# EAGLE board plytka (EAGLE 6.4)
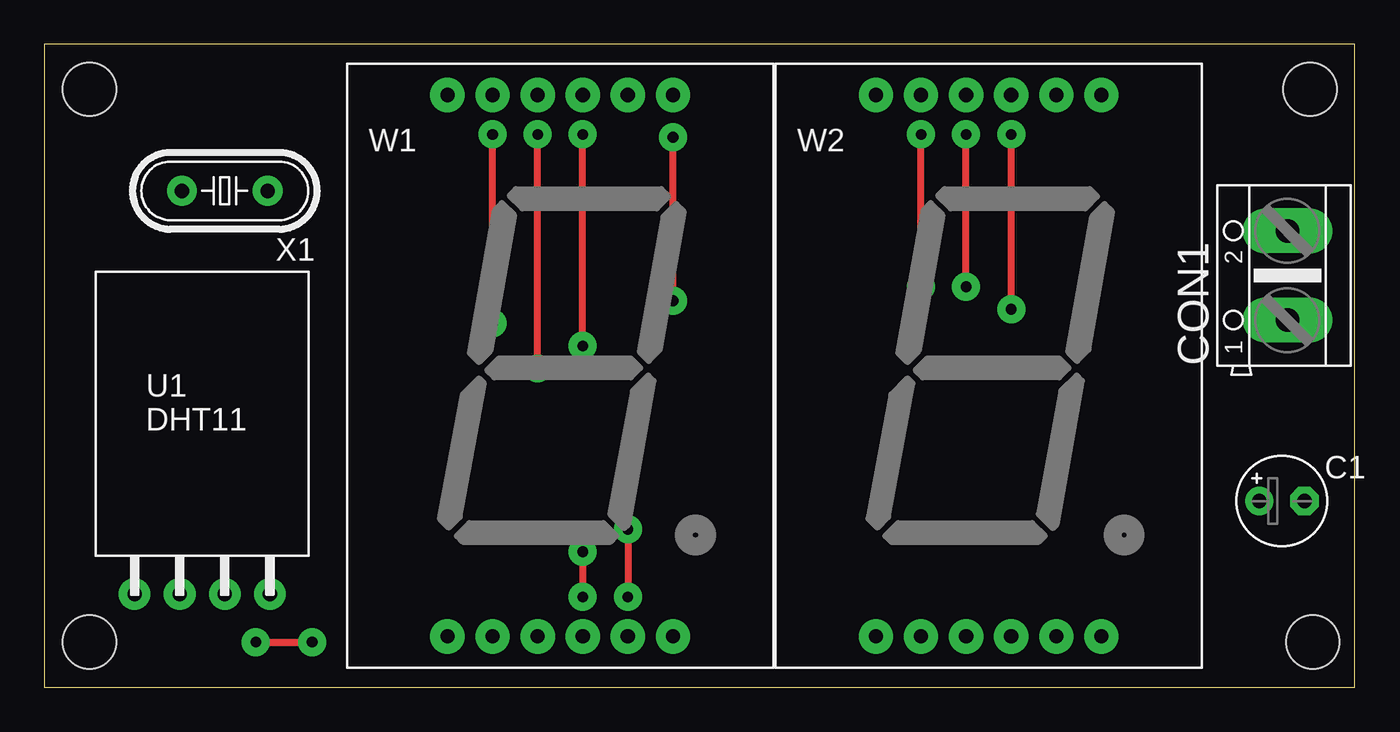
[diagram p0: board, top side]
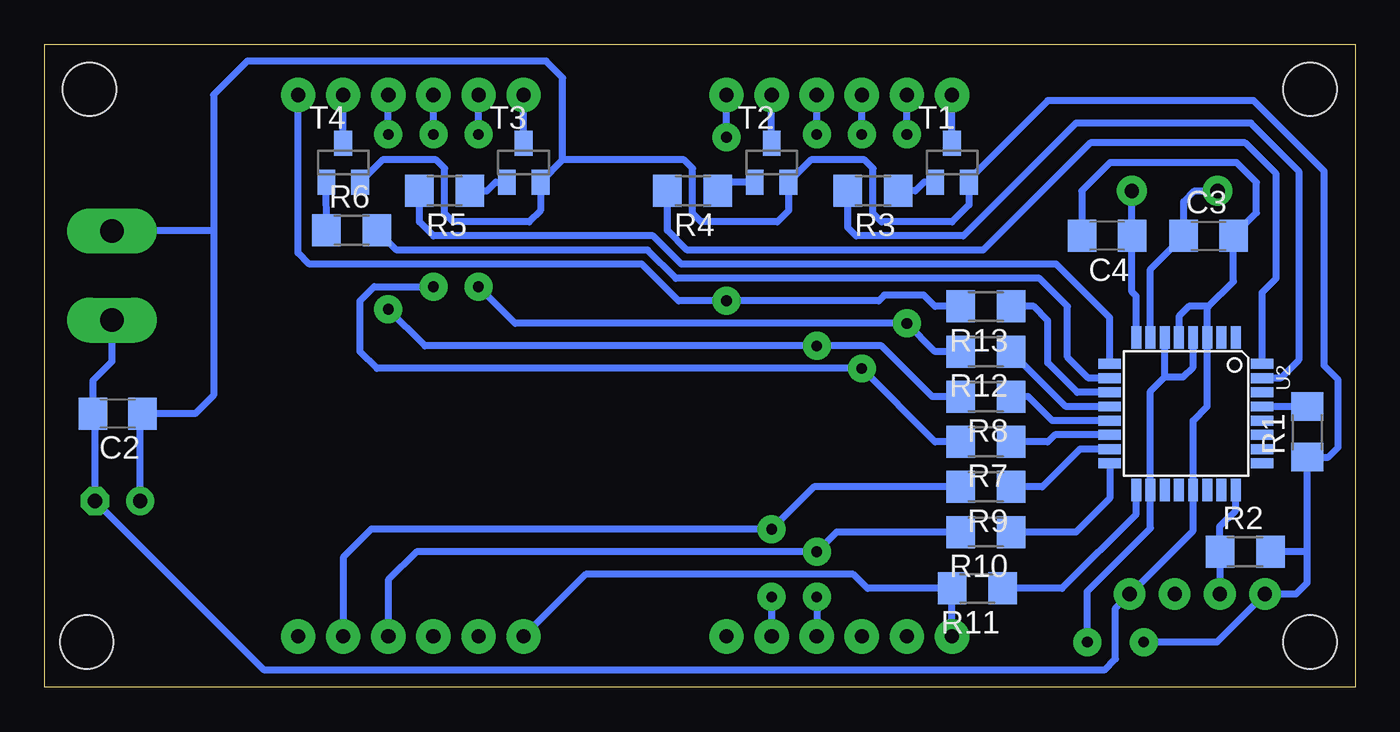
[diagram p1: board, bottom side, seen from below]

Size 73.81 x 36.19 mm. Coordinates in mm from the lower left corner, seen from the top.
Outline: 0,0 73.81,0 73.81,36.19 0,36.19 0,0
Copper layers (1*16): Top 0.035mm / dielectric 1.5mm / Bottom 0.035mm
Design rules "default": minimum track width 10mil, minimum drill 24mil, track to track 8mil, track to pad 8mil, pad to pad 8mil, via to via 8mil, smd to smd 8mil, copper to edge 40mil, drill to drill 8mil, minimum pad ring 10mil, minimum via ring 8mil, stop-mask expansion 4mil, vias tented up to drill 0mil, thermal gap 10mil
Holes 3 mm at 71.28,33.66 71.44,2.54 2.54,33.66 2.54,2.54

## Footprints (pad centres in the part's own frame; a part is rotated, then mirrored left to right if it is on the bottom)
E2,5-5 = drill 0.813 pad 1.6: + -1.27,0 | drill 0.813 pad 1.6 octagon: - 1.27,0
C1206 = smd 1.6 x 1.8: 1 -1.4,0; 2 1.4,0
AK500/2 = drill 1.321 pad 2.54 long: 1 -2.515,0; 2 2.515,0
R1206 = smd 1.6 x 1.803: 1 -1.422,0; 2 1.422,0
SOT23-BEC = smd 1 x 1.4: B -0.95,-1.1; C 0,1.1; E 0.95,-1.1
DHT11 = drill 0.8 pad 1.778: 1 -3.81,-10.16; 2 -1.27,-10.16; 3 1.27,-10.16; 4 3.81,-10.16
TQFP32-08 = smd 1.27 x 0.559: 1 -4.293,2.8; 2 -4.293,2; 3 -4.293,1.2; 4 -4.293,0.4; 5 -4.293,-0.4; 6 -4.293,-1.2; 7 -4.293,-2; 8 -4.293,-2.8; 17 4.293,-2.8; 18 4.293,-2; 19 4.293,-1.2; 20 4.293,-0.4; 21 4.293,0.4; 22 4.293,1.2; 23 4.293,2; 24 4.293,2.8 | smd 0.559 x 1.27: 9 -2.8,-4.293; 10 -2,-4.293; 11 -1.2,-4.293; 12 -0.4,-4.293; 13 0.4,-4.293; 14 1.2,-4.293; 15 2,-4.293; 16 2.8,-4.293; 25 2.8,4.293; 26 2,4.293; 27 1.2,4.293; 28 0.4,4.293; 29 -0.4,4.293; 30 -1.2,4.293; 31 -2,4.293; 32 -2.8,4.293
LED1-AS-10016 = drill 0.8 pad 1.93: 1 -6.35,-15.24; 2 -3.81,-15.24; 3 -1.27,-15.24; 4 1.27,-15.24; 5 3.81,-15.24; 6 6.35,-15.24; 7 6.35,15.24; 8 3.81,15.24; 9 1.27,15.24; 10 -1.27,15.24; 11 -3.81,15.24; 12 -6.35,15.24
HC49/S = drill 0.813 pad 1.676: 1 -2.413,0; 2 2.413,0

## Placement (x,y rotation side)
C1  10u  [E2,5-5]  69.69,10.48 0 top
C2  100n  [C1206]  69.69,15.4 180 bottom
C3  33p  [C1206]  8.26,25.4 0 bottom
C4  33p  [C1206]  13.97,25.4 180 bottom
CON1  [AK500/2]  70.01,23.18 90 top
R1  10k  [R1206]  2.7,14.37 90 bottom
R2  4k7  [R1206]  6.19,7.62 0 bottom
R3  3k3  [R1206]  27.15,27.94 180 bottom
R4  3k3  [R1206]  37.31,27.94 180 bottom
R5  3k3  [R1206]  51.28,27.94 180 bottom
R6  3k3  [R1206]  56.52,25.72 0 bottom
R7  150  [R1206]  20.8,13.81 180 bottom
R8  150  [R1206]  20.8,16.35 180 bottom
R9  [R1206]  20.8,11.27 180 bottom
R10  [R1206]  20.8,8.73 180 bottom
R11  [R1206]  21.27,5.56 180 bottom
R12  150  [R1206]  20.8,18.89 180 bottom
R13  150  [R1206]  20.8,21.43 180 bottom
T1  BC857  [SOT23-BEC]  22.7,29.53 0 bottom
T2  BC857  [SOT23-BEC]  32.86,29.53 0 bottom
T3  BC857  [SOT23-BEC]  46.83,29.53 0 bottom
T4  BC857  [SOT23-BEC]  56.99,29.53 0 bottom
U1  DHT11  [DHT11]  8.89,15.4 0 top
U2  ATmega8  [TQFP32-08]  9.53,15.4 270 bottom
W1  [LED1-AS-10016]  29.05,18.1 0 top
W2  [LED1-AS-10016]  53.18,18.1 0 top
X1  4MHz  [HC49/S]  10.16,27.94 180 top

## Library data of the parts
C1-C4 R1-R13 = rcl
CON1 = con-ptr500
T1-T4 = transistor
U1 = sensors
U2 = atmel
W1 W2 = display-hp
X1 = crystal

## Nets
A: R7.1 U2.14
B: R8.1 U2.13
C: R9.1 U2.15
CZ: R2.1 U1.2 U2.24
D: R10.1 U2.16
E: R11.1 U2.17
F: R12.1 U2.12
G: R13.1 U2.11
GND: C1.- C2.2 C3.2 C4.2 CON1.1 U1.4 U2.3 U2.5 U2.21
N$1: R7.2 W1.10 W2.10
N$2: R8.2 W1.9 W2.9
N$3: R9.2 W1.5 W2.5
N$4: R10.2 W1.4 W2.4
N$5: R11.2 W1.1 W2.1
N$6: R12.2 W1.11 W2.11
N$7: R13.2 W1.7 W2.7
N$8: T1.C W1.12
N$9: T2.C W1.8
N$10: T3.C W2.12
N$11: T4.C W2.8
N$12: R4.1 T2.B
N$13: R5.1 T3.B
N$14: R6.1 T4.B
N$19: R3.1 T1.B
N$27: R1.2 U2.29
N$33: C3.1 U2.7 X1.2
N$34: C4.1 U2.8 X1.1
T1: R3.2 U2.31
T2: R4.2 U2.32
T3: R5.2 U2.9
T4: R6.2 U2.10
VCC: C1.+ C2.1 CON1.2 R1.1 R2.2 T1.E T2.E T3.E T4.E U1.1 U2.4 U2.6 U2.18

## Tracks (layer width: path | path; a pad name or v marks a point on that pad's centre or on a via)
A
  Bottom 0.406: U2.14 16.92,14.2 17.3,13.81 R7.1 | R7.1
B
  Bottom 0.406: U2.13 17.06,15 18.41,16.35 R8.1 | R8.1
C
  Bottom 0.406: U2.15 15.49,13.4 17.62,11.27 R9.1
CZ
  Bottom 0.406: U1.2 | U1.2 7.62,7.3 R2.1 7.62,9.05 6.72,9.94 U2.24
D
  Bottom 0.406: U2.16 13.82,10.63 15.72,8.73 R10.1 | R10.1
E
  Bottom 0.406: U2.17 12.32,9.74 16.51,5.56 R11.1
F
  Bottom 0.406: R12.1 | U2.12 16.28,15.8 R12.1
G
  Bottom 0.406: R13.1 | U2.11 15.65,16.6 17.3,18.26 17.3,20.64 18.1,21.43 R13.1
GND
  Bottom 0.406: CON1.1 70.01,18.34 71.09,17.25 C2.2 70.96,15.27 C1.- 61.44,0.95 14.13,0.95 13.49,1.59 13.49,4.45 U1.4 9.12,8.81 U2.21 9.12,15.01 8.32,15.8 U2.3 8.32,21.36 8.26,21.43 | U2.5 9.93,20.87 9.37,21.43 8.26,21.43 | C4.2 15.4,25.59 15.4,27.94 13.81,29.53 6.67,29.53 5.56,28.42 5.56,26.7 C3.2 6.86,22.83 8.26,21.43
N$1  (via drill 0.6 pad 1.57)
  Top 0.406: v51.91,22.54 v51.91,31.11 | v27.78,17.94 v27.78,31.11
  Bottom 0.406: v51.91,31.11 W2.10 | v27.78,31.11 W1.10 | v51.91,22.54 55.24,22.54 56.04,21.75 56.04,18.89 55.09,17.94 v27.78,17.94 23.65,13.81 R7.2
N$2  (via drill 0.6 pad 1.57)
  Top 0.406: v30.32,19.21 v30.32,31.11 | v54.45,21.27 v54.45,31.11
  Bottom 0.406: v30.32,31.11 W1.9 | v54.45,31.11 W2.9 | v30.32,19.21 52.39,19.21 v54.45,21.27 | v30.32,19.21 | v30.32,19.21 26.67,19.21 23.81,16.35 R8.2 | R8.2
N$3  (via drill 0.6 pad 1.57)
  Top 0.406: v32.86,8.89 v32.86,5.08
  Bottom 0.406: v32.86,5.08 W1.5 | W2.5 56.99,7.3 55.4,8.89 v32.86,8.89 30.48,11.27 R9.2
N$4  (via drill 0.6 pad 1.57)
  Top 0.406: v30.32,7.62 v30.32,5.08
  Bottom 0.406: v30.32,5.08 W1.4 | W2.4 54.45,6.03 52.86,7.62 v30.32,7.62 29.21,8.73 R10.2
N$5
  Bottom 0.406: W1.1 22.7,5.55 R11.2 27.46,5.56 28.26,6.35 43.34,6.35 W2.1
N$6  (via drill 0.6 pad 1.57)
  Top 0.406: v25.24,20.48 v25.24,31.11 | v49.37,22.54 v49.37,31.11
  Bottom 0.406: v25.24,31.11 W1.11 | v49.37,31.11 W2.11 | v49.37,22.54 47.31,20.48 v25.24,20.48 23.65,18.89 R12.2
N$7  (via drill 0.6 pad 1.57)
  Top 0.406: v35.4,21.75 v35.4,30.96
  Bottom 0.406: v35.4,30.96 W1.7 | W2.7 59.53,24.45 58.9,23.81 40.16,23.81 38.1,21.75 v35.4,21.75 26.83,21.75 26.67,21.91 26.51,22.07 24.29,22.07 23.65,21.43 R13.2 | R13.2
N$8
  Bottom 0.406: T1.C W1.12
N$9
  Bottom 0.406: T2.C W1.8
N$10
  Bottom 0.406: T3.C W2.12
N$11
  Bottom 0.406: T4.C W2.8
N$12
  Bottom 0.406: T2.B 35.4,28.43 R4.1
N$13
  Bottom 0.406: T3.B 48.41,28.43 48.9,27.94 R5.1 | R5.1
N$14
  Bottom 0.406: R6.1 T4.B
N$19
  Bottom 0.406: T1.B 24.28,28.43 24.77,27.94 R3.1
N$27
  Bottom 0.406: R1.2 5.22,15.79 U2.29
N$33
  Bottom 0.406: X1.2 9.05,27.94 9.65,27.33 C3.1 11.53,23.53 U2.7
N$34
  Bottom 0.406: X1.1 C4.1 12.57,22.25 12.32,22.01 U2.8
T1
  Bottom 0.406: R3.2 28.57,25.87 28.1,25.4 22.07,25.4 15.72,31.75 5.87,31.75 3.17,29.05 3.17,18.41 4.19,17.4 U2.31
T2
  Bottom 0.406: U2.32 5.24,22.23 4.45,23.02 4.45,28.89 6.19,30.64 14.92,30.64 20.95,24.61 37.62,24.61 38.73,25.71 R4.2
T3
  Bottom 0.406: U2.9 13.82,20.8 16.83,23.81 37.94,23.81 39.53,25.4 51.91,25.4 52.7,26.19 R5.2
T4
  Bottom 0.406: U2.10 15.02,17.4 16.19,18.57 16.19,21.43 17.78,23.02 38.26,23.02 39.85,24.61 53.98,24.61 R6.2
VCC  (via drill 0.6 pad 1.57)
  Top 0.406: v11.91,2.54 v15.08,2.54
  Bottom 0.406: T1.E 21.75,27.15 22.7,26.19 26.67,26.19 27.15,26.67 27.15,29.21 27.62,29.69 30.65,29.69 T2.E 31.91,28.11 31.91,26.83 32.54,26.19 36.83,26.19 37.31,26.67 37.31,29.21 37.78,29.69 44.62,29.69 | T1.E | 56.04,28.57 T4.E 54.78,29.69 51.75,29.69 51.28,29.21 51.28,26.67 50.8,26.19 46.51,26.19 45.88,26.83 T3.E 44.62,29.69 | 44.62,29.69 44.62,34.3 45.56,35.24 62.39,35.24 64.29,33.34 64.29,25.69 | v11.91,2.54 7.78,2.54 U1.1 | 64.29,25.69 CON1.2 | 64.29,25.69 64.29,16.43 65.33,15.4 C2.1 68.42,15.27 C1.+ | R1.1 | 2.7,7.62 R1.1 | 2.7,7.62 2.7,5.87 3.33,5.24 U1.1 | U1.1 | 2.7,7.62 R2.2 | R1.1 1.5,12.95 0.95,13.49 0.95,17.3 1.75,18.1 1.75,29.05 5.71,33.02 17.3,33.02 21.75,28.57 T1.E | U2.4 9.12,18.02 9.68,17.46 10.72,17.46 | 10.72,17.46 U2.6 | 10.72,17.46 11.53,16.66 U2.18 11.53,8.95 15.08,5.4 v15.08,2.54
